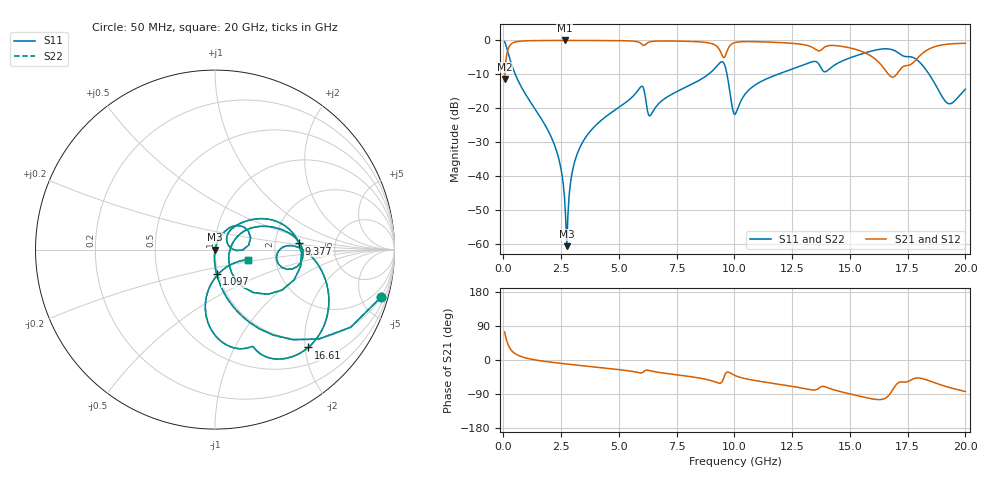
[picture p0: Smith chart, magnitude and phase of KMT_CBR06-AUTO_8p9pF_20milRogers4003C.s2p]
! Data measured by Modelithics Inc. support@modelithics.com 813-866-6335
! KEMET CBR06-AUTO 8.9pF, Pad Width= 0.851mm, Pad Length= 0.64mm, Pad Gap= 0.62mm, 20mil Rogers 4003C substrate Data, January 2022
# hz S ma R 50
! 2 Port Network Data from SP1.SP block
! freq  magS11  angS11  magS21  angS21  magS12  angS12  magS22  angS22
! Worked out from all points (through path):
!   401 points, 50 MHz to 20 GHz, reference 50 ohm
!   highest |S21| = -0.01 dB at 2.643 GHz (marker M1); lowest = -11.3 dB at 50 MHz (marker M2)
!   group delay of S21, straight-line fit = 13.2 ps
!   lowest |S11| = -60.5 dB at 2.743 GHz (marker M3), VSWR 1.00, Z = 50.1 + j0.00152 ohm
!   |S11| at or under -10 dB: 514.8 MHz to 8.866 GHz (8.351 GHz wide, 178 % of centre); 9.679 GHz to 11.86 GHz (2.181 GHz wide, 20.3 % of centre); 18.43 GHz to end of sweep
!   |S22| runs from -60.5 to -0.3 dB; largest |S21 - S12| = 0
!   S11 on the Smith chart (normalised r, x): 50 MHz: 0.98, -7.02; 1.097 GHz: 0.98, -0.27; 9.377 GHz: 2.75, +0.24; 16.61 GHz: 0.82, -2.07; 20 GHz: 1.44, -0.17
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5e7  0.9625 -15.9  0.2711 74.1  0.2711 74.1  0.9625 -15.9
3.99125e8  0.3994 -67.9  0.9162 22.0  0.9162 22.0  0.3994 -67.9
1.097375e9  0.1356 -86.2  0.9901 3.5  0.9901 3.5  0.1356 -86.2
2.2445e9  0.02687 -95.4  0.9987 -7.2  0.9987 -7.2  0.02687 -95.4
2.6435e9  0.004924 -89.4  0.999 -10.0  0.999 -10.0  0.004924 -89.4
2.74325e9  0.0009413 0.9  0.999 -10.7  0.999 -10.7  0.0009413 0.9
3.0425e9  0.01454 73.5  0.9988 -12.7  0.9988 -12.7  0.01454 73.5
3.391625e9  0.03023 73.1  0.9984 -14.9  0.9984 -14.9  0.03023 73.1
5.93525e9  0.2062 36.1  0.9111 -34.2  0.9111 -34.2  0.2062 36.1
6.33425e9  0.07752 26.3  0.9526 -28.1  0.9526 -28.1  0.07752 26.3
6.73325e9  0.1187 51.3  0.9805 -32.8  0.9805 -32.8  0.1187 51.3
9.376625e9  0.4697 4.2  0.7083 -61.2  0.7083 -61.2  0.4697 4.2
9.626e9  0.384 -40.5  0.617 -34.5  0.617 -34.5  0.384 -40.5
1.0025e10  0.0819 -6.5  0.931 -40.9  0.931 -40.9  0.0819 -6.5
1.092275e10  0.224 31.4  0.9581 -54.5  0.9581 -54.5  0.224 31.4
1.336662e10  0.4857 1.0  0.7926 -78.9  0.7926 -78.9  0.4857 1.0
1.50125e10  0.5551 -5.7  0.7751 -89.7  0.7751 -89.7  0.5551 -5.7
1.66085e10  0.753 -46.4  0.3375 -97.7  0.3375 -97.7  0.753 -46.4
1.670825e10  0.7473 -50.3  0.3071 -91.4  0.3071 -91.4  0.7473 -50.3
1.825438e10  0.3861 -96.8  0.6906 -51.2  0.6906 -51.2  0.3861 -96.8
1.925188e10  0.1181 -63.4  0.8823 -71.5  0.8823 -71.5  0.1181 -63.4
2e10  0.1919 -17.0  0.9063 -83.1  0.9063 -83.1  0.1919 -17.0
